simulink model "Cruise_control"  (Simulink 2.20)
settings: Solver=FixedStepDiscrete  StartTime=0.0  StopTime=10  FixedStep=0.02  RelTol=1e-3  AbsTol=1e-6

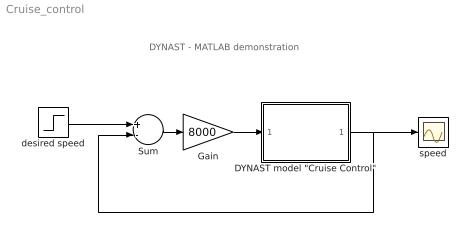
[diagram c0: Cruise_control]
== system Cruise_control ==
  note: DYNAST - MATLAB demonstration
  "DYNAST model \"Cruise Control\"" : Subsystem
  Gain : Gain  Gain=8000
  Sum : Sum  Inputs=+-
  desired speed : Step  Time=0  Before=0  After=10
  speed : Scope
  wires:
  Gain/1 -> "DYNAST model \"Cruise Control\""/1(u)
  Sum/1 -> Gain/1
  "DYNAST model \"Cruise Control\""/1("v ") -> speed/1, Sum/2
  desired speed/1 -> Sum/1

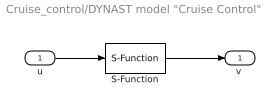
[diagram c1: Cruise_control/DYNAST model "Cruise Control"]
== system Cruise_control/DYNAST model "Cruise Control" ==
  u : Inport  Port=1  PortWidth=-1  SampleTime=-1
  S-Function : S-Function  FunctionName=dynPlantL  Parameters='%DYNAST%\examples\control\CruiseControl.prb',0.02  PortCounts=[]  SFunctionModules=''
  "v " : Outport  Port=1
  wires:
  S-Function/1 -> "v "/1
  u/1 -> S-Function/1
